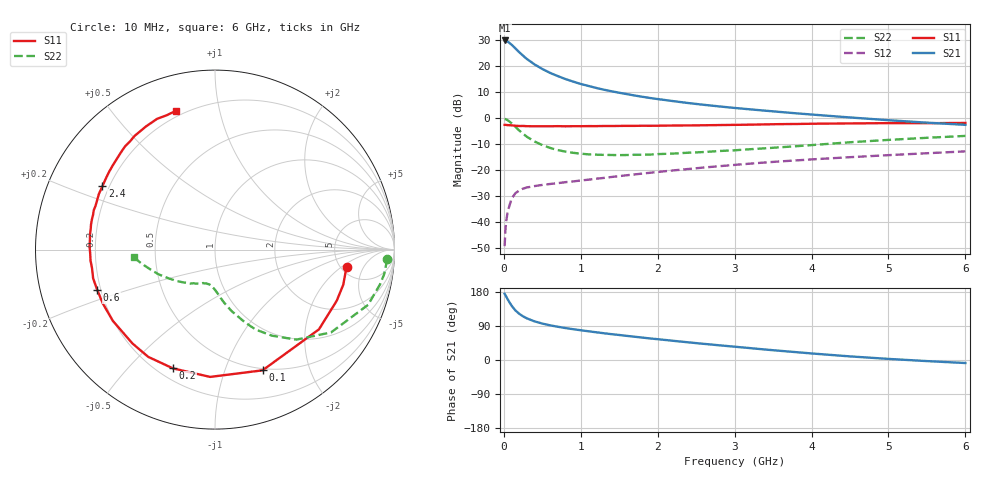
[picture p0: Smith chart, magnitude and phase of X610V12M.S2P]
! SIEMENS Small Signal Semiconductors
! BFP193W
! Si NPN RF Bipolar Junction Transistor in SOT343
! VCE = 10 V  IC = 12 mA
! Common Emitter S-Parameters:  April 1994
# GHz  S  MA  R  50
!  f  S11  S21  S12  S22
! GHz  MAG  ANG  MAG  ANG  MAG  ANG  MAG  ANG
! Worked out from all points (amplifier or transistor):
!   40 points, 10 MHz to 6 GHz, reference 50 ohm
!   highest |S21| = 29.7 dB at 10 MHz (marker M1)
!   |S21| within 3 dB of that: start of sweep to 149.1 MHz
!   unconditionally stable (mu >= 1): 1.298 GHz to 4.467 GHz
!   at 200 MHz: K = 0.25, MSG = 26.5 dB, |S12| = -27.8 dB
!   at 1.5 GHz: K = 1.05, MAG = 14.6 dB, |S12| = -22.3 dB
!   at 6 GHz: K = 0.94, MSG = 5.1 dB, |S12| = -12.8 dB
!   S11 on the Smith chart (normalised r, x): 10 MHz: 5.62, -2.39; 100 MHz: 0.48, -1.36; 200 MHz: 0.26, -0.67; 600 MHz: 0.19, -0.16; 2.4 GHz: 0.17, +0.25; 6 GHz: 0.17, +0.74
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0.01  0.739 -7.5  30.59 174.6  0.0035 77.7  0.961 -3.2
0.02  0.741 -15.3  30.56 171.5  0.0069 77.3  0.9527 -8.2
0.03  0.7356 -22.8  30.16 167.7  0.0103 77.7  0.9392 -12.0
0.05  0.73 -37.5  29.1 159.9  0.0161 71.5  0.9071 -19.8
0.1  0.7229 -68.5  25.43 143.6  0.0283 58.6  0.7944 -35.5
0.15  0.7098 -92.2  21.59 130.9  0.0362 49.0  0.676 -47.9
0.2  0.702 -109.5  18.21 121.9  0.0408 43.0  0.5752 -56.5
0.25  0.704 -121.9  15.63 115.1  0.0443 39.0  0.5004 -63.0
0.3  0.6964 -131.4  13.49 109.8  0.0467 36.5  0.4362 -67.8
0.4  0.694 -145.1  10.6 101.9  0.0496 34.0  0.3545 -74.9
0.5  0.6933 -154.3  8.684 96.1  0.0522 33.3  0.3024 -80.0
0.6  0.6935 -161.2  7.32 91.5  0.0544 33.8  0.2675 -83.8
0.8  0.6929 -171.4  5.576 84.3  0.0589 35.5  0.227 -89.5
1.1  0.6992 178.7  4.114 75.8  0.0658 38.9  0.2009 -96.2
1.3  0.7016 173.3  3.485 70.6  0.0711 41.0  0.1965 -99.9
1.6  0.7061 166.2  2.866 63.6  0.08 43.4  0.1953 -105.0
2.2  0.7173 154.4  2.107 50.7  0.0989 45.7  0.2081 -115.5
2.4  0.7197 150.6  1.931 46.6  0.1055 45.9  0.2163 -118.6
3.2  0.7448 137.2  1.465 31.4  0.1334 44.7  0.252 -133.2
4.5  0.7867 119.2  1.024 9.5  0.1774 39.6  0.3428 -156.2
5.5  0.7953 109.9  0.814 -2.9  0.2112 34.9  0.4173 -169.3
6  0.8036 105.6  0.739 -8.0  0.2293 32.6  0.4533 -174.5
